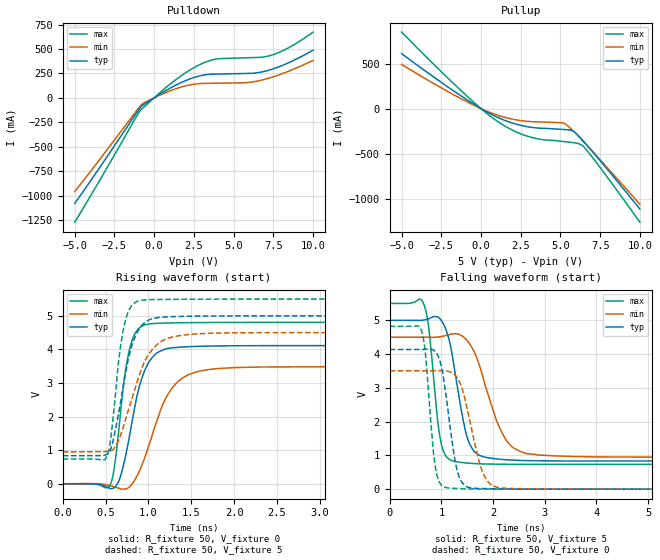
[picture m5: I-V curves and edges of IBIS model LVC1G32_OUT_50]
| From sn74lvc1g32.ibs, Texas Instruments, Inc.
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[Model]   LVC1G32_OUT_50
Model_type  Output
Vref =   0.0
Rref =   500
Cref =   50p
Vmeas =   2.5
| variable   typ   min   max
C_comp   8.09pF   5.98pF   11.15pF
| C_pullup   7.98pF   6.07pF   9.05pF
| C_pulldown   8.19pF   5.98pF   11.15pF
[Temperature Range]   40   100   -40
| Ambient temperature   25   85   -40
[Voltage range]   5   4.5   5.5
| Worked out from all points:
|   slope of the pulldown table from 0 to 0.75 V, typ, clamps not added: 9.97 ohm
|   slope of the pullup table from 0 to 0.75 V, typ, clamps not added: 10.3 ohm
|   rising waveform, R_fixture 50, V_fixture 0: 20-80 % time 211ps typ, 314ps min, 139ps max; typ from 0 V to 4.11 V
|   rising waveform, R_fixture 50, V_fixture 5: 20-80 % time 194ps typ, 283ps min, 129ps max; typ from 0.835 V to 5 V
|   falling waveform, R_fixture 50, V_fixture 5: 20-80 % time 288ps typ, 469ps min, 185ps max; typ from 5 V to 0.835 V
|   falling waveform, R_fixture 50, V_fixture 0: 20-80 % time 229ps typ, 317ps min, 155ps max; typ from 4.13 V to 0 V
[Pulldown]
| LVC1G32_OUT_50
|   Voltage   I(typ)   I(min)   I(max)
-5V       -1.081A    -958.7mA   -1.272A
-930mV    -112.8mA   -95.57mA   -141.9mA
-615mV    -65.29mA   -48.71mA   -90.86mA
1.06V     103.7mA    74.73mA    147.4mA
2.29V     195.8mA    133.5mA    288.4mA
3.355V    239mA      148.3mA    373mA
4.1V      243.6mA    149.9mA    400.8mA
5.83V     249.3mA    155.5mA    409.8mA
6.545V    257.6mA    173.1mA    413.3mA
7.3V      286.7mA    205mA      432.2mA
8.52V     363.3mA    276.1mA    517mA
10V       487.1mA    382.2mA    672.5mA
[Pullup]
| LVC1G32_OUT_50
|   Voltage   I(typ)   I(min)   I(max)
-5V       610.5mA    490.7mA    849.3mA
-1.265V   141.7mA    110.6mA    201.1mA
150mV     -15.75mA   -12.02mA   -22.71mA
1.045V    -97.45mA   -73.04mA   -142.5mA
2.015V    -162.5mA   -118.6mA   -242mA
3.01V     -203.9mA   -143mA     -311.3mA
3.86V     -218.8mA   -148.7mA   -344.2mA
5.285V    -233.1mA   -167.8mA   -367.4mA
5.825V    -250.9mA   -252.6mA   -378.1mA
6.475V    -367.7mA   -371.7mA   -425.3mA
7.675V    -615.1mA   -602.6mA   -696.3mA
10V       -1.115A    -1.063A    -1.261A
[Ramp]
| LVC1G32_OUT_50
| variable   typ   min   max
dV/dt_r   2.56/2.22E-10   2.18/3.29E-10   2.95/1.45E-10
dV/dt_f   2.57/3.01E-10   2.19/5.06E-10   2.94/1.98E-10
R_load = 50
[Rising Waveform]
| LVC1G32_OUT_50
R_fixture =   50
C_fixture =   0
L_fixture =   0
V_fixture =   0
V_fixture_min = 0
V_fixture_max = 0
|   Time   V(typ)   V(min)   V(max)
0s        -15.13uV   -63.34uV   -40.93nV
545ps     -134.3mV   -51.44mV   -79.63mV
595ps     -126.7mV   -86.64mV   379.6mV
665ps     154.8mV    -143.6mV   1.879V
795ps     1.653V     -48.09mV   4.157V
940ps     3.267V     663.4mV    4.714V
1.12ns    3.928V     2.034V     4.78V
1.455ns   4.08V      3.232V     4.797V
2.32ns    4.113V     3.477V     4.806V
50ns      4.113V     3.48V      4.806V
[Rising Waveform]
| LVC1G32_OUT_50
R_fixture =   50
C_fixture =   0
L_fixture =   0
V_fixture =   5
V_fixture_min = 4.5
V_fixture_max = 5.5
|   Time   V(typ)   V(min)   V(max)
0s        835.1mV    949.5mV    736.2mV
500ps     859.5mV    960.5mV    750mV
585ps     1.258V     1.01V      1.908V
665ps     2.295V     1.383V     3.92V
740ps     3.395V     1.978V     4.943V
860ps     4.468V     2.974V     5.422V
1.02ns    4.894V     3.914V     5.483V
1.295ns   4.979V     4.38V      5.492V
2.095ns   4.999V     4.498V     5.5V
50ns      5V         4.5V       5.5V
[Falling Waveform]
| LVC1G32_OUT_50
R_fixture =   50
C_fixture =   0
L_fixture =   0
V_fixture =   5
V_fixture_min = 4.5
V_fixture_max = 5.5
|   Time   V(typ)   V(min)   V(max)
0s        5V         4.5V       5.5V
670ps     5.01V      4.499V     5.443V
755ps     5.046V     4.497V     4.79V
925ps     5.101V     4.504V     2.069V
1.015ns   4.962V     4.524V     1.241V
1.16ns    4.364V     4.58V      876.4mV
1.59ns    1.221V     4.196V     762.5mV
2.285ns   868.5mV    1.389V     737mV
3.185ns   835.4mV    985.2mV    735.4mV
50ns      835.1mV    949.5mV    736.2mV
[Falling Waveform]
| LVC1G32_OUT_50
R_fixture =   50
C_fixture =   0
L_fixture =   0
V_fixture =   0
V_fixture_min = 0
V_fixture_max = 0
|   Time   V(typ)   V(min)   V(max)
0s        4.135V     3.505V     4.823V
610ps     4.136V     3.505V     4.713V
690ps     4.143V     3.505V     4.04V
895ps     4.056V     3.507V     564.1mV
1.015ns   3.507V     3.51V      101.5mV
1.175ns   1.771V     3.47V      29.27mV
1.415ns   166.2mV    2.912V     13.58mV
1.81ns    17.57mV    461.8mV    3.46mV
2.24ns    5.976mV    25.74mV    557.5uV
50ns      -13.59uV   -62.53uV   2.503uV
